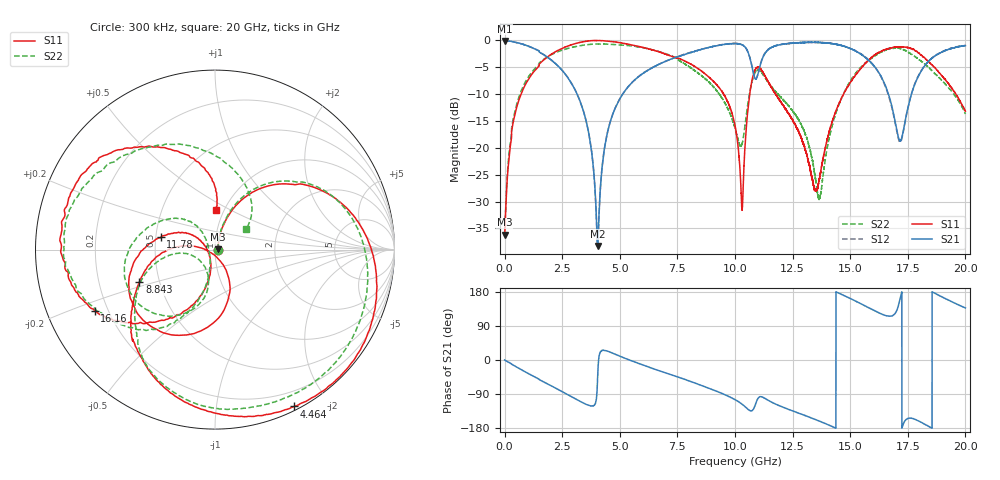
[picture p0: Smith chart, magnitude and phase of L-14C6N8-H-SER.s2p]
!{L-14C6N8}
!Johanson Technology Inc.
!www.johansontechnology.com
!Test Board Conditions:
!Substrate Type  RO4350B
!Substrate Thickness  20 mil
!Substrate Dk  3.66
!TL Type: GCPW
!TL Trace Width  36 mil
!TL Gap  12 mil
!Electrode orientation  Horizontal
!DUT TOPOLOGY	SERIES
!Mounting Pad LxW  26x36 mil
! Created Sun Jun 20 12:59:06 2021
# hz S ma R 50
! 2 Port Network Data from SP1.SP block
! freq  magS11  angS11  magS21  angS21  magS12  angS12  magS22  angS22
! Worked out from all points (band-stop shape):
!   20001 points, 300 kHz to 20 GHz, reference 50 ohm
!   highest |S21| = -0.14 dB at 12.3 MHz (marker M1); lowest = -38.3 dB at 4.039 GHz (marker M2)
!   |S21| within 3 dB of the highest: 7.465 GHz to 10.63 GHz (3.169 GHz wide, 35 % of centre); 11.22 GHz to 15.63 GHz (4.41 GHz wide, 32.9 % of centre)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
!   lowest |S11| = -36.1 dB at 2.3 MHz (marker M3), VSWR 1.03, Z = 51.6 + j0.106 ohm
!   |S11| at or under -10 dB: start of sweep to 717.5 MHz; 9.503 GHz to 10.64 GHz (1.138 GHz wide, 11.3 % of centre); 11.76 GHz to 14.71 GHz (2.958 GHz wide, 22.4 % of centre)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
!   |S22| runs from -36.5 to -0.7 dB; largest |S21 - S12| = 0.014
!   S11 on the Smith chart (normalised r, x): 300 kHz: 1.03, -0.00; 4.464 GHz: 0.04, -1.62; 8.843 GHz: 0.38, -0.18; 11.78 GHz: 0.53, +0.08; 16.16 GHz: 0.15, -0.24; 20 GHz: 0.92, +0.42
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300000  0.01565 -2.4  0.9844 0.0  0.9844 0.1  0.01491 -1.9
2300000  0.01559 3.8  0.9843 -0.1  0.9845 -0.1  0.01573 4.1
1.23e7  0.01682 19.2  0.9844 -0.5  0.9838 -0.5  0.01709 20.3
3.173e8  0.1478 70.7  0.9674 -11.5  0.9677 -11.5  0.1589 71.2
7.773e8  0.339 60.0  0.9176 -27.4  0.918 -27.4  0.3605 60.2
3.3343e9  0.9594 -23.5  0.2496 -110.9  0.2504 -110.8  0.8922 -21.8
4.0393e9  0.9923 -48.8  0.01219 -45.5  0.01216 -45.5  0.9214 -47.1
4.4643e9  0.9789 -63.2  0.1382 23.3  0.1387 23.2  0.9171 -61.0
6.6673e9  0.7834 -116.3  0.5922 -27.5  0.5933 -27.2  0.7867 -114.5
8.8433e9  0.4588 -156.8  0.8529 -74.0  0.8535 -74.1  0.4127 -160.7
1.00003e10  0.1613 172.7  0.9306 -104.6  0.9313 -104.6  0.1525 -170.5
1.03013e10  0.02668 -131.6  0.9068 -116.3  0.9062 -116.3  0.1073 -125.2
1.08393e10  0.5092 -110.2  0.4581 -125.0  0.4612 -125.1  0.4814 -131.6
1.17793e10  0.3101 167.1  0.8891 -116.8  0.8901 -116.9  0.3293 150.0
1.33343e10  0.05317 164.2  0.955 -153.4  0.9539 -153.4  0.08067 131.2
1.36723e10  0.05246 -121.5  0.9506 -161.5  0.9494 -161.5  0.03447 -162.0
1.45543e10  0.2688 -107.6  0.8973 175.2  0.8981 175.2  0.2654 -106.5
1.61563e10  0.7522 -153.0  0.5319 126.9  0.5321 127.2  0.7354 -151.8
1.66673e10  0.8278 -171.0  0.3127 116.0  0.3035 116.5  0.8343 -172.9
1.71803e10  0.8631 165.8  0.1163 164.7  0.1133 164.8  0.8355 163.0
1.80193e10  0.7462 130.7  0.4888 -162.6  0.4932 -161.6  0.6496 116.5
2e10  0.2183 88.7  0.89 137.4  0.8896 137.4  0.2057 33.2
